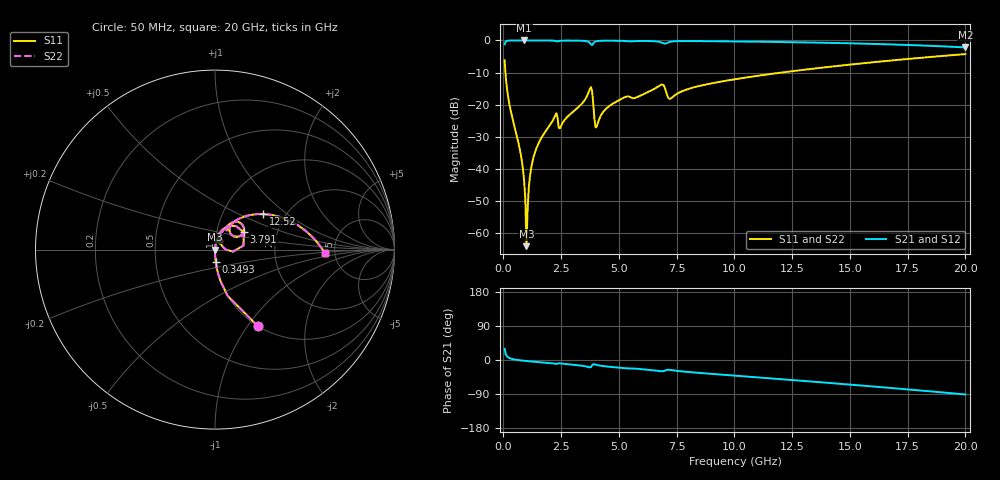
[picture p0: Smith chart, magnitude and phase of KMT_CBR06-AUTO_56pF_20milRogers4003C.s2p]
! Data measured by Modelithics Inc. support@modelithics.com 813-866-6335
! KEMET CBR06-AUTO 56pF, Pad Width= 0.851mm, Pad Length= 0.64mm, Pad Gap= 0.62mm, 20mil Rogers 4003C substrate Data, January 2022
# hz S ma R 50
! 2 Port Network Data from SP1.SP block
! freq  magS11  angS11  magS21  angS21  magS12  angS12  magS22  angS22
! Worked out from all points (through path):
!   401 points, 50 MHz to 20 GHz, reference 50 ohm
!   highest |S21| = 0.00 dB at 897.9 MHz (marker M1); lowest = -2.2 dB at 20 GHz (marker M2)
!   group delay of S21, straight-line fit = 12.8 ps
!   lowest |S11| = -64.0 dB at 997.6 MHz (marker M3), VSWR 1.00, Z = 50 - j0.0408 ohm
!   |S11| at or under -10 dB: 86.67 MHz to 12.03 GHz (11.95 GHz wide, 197 % of centre)
!   |S22| runs from -64.0 to -4.2 dB; largest |S21 - S12| = 0
!   S11 on the Smith chart (normalised r, x): 50 MHz: 1.00, -1.13; 349.2 MHz: 1.00, -0.14; 3.791 GHz: 1.35, +0.27; 12.52 GHz: 1.54, +0.69; 20 GHz: 4.15, -0.28
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5e7  0.4912 -60.7  0.8707 29.3  0.8707 29.3  0.4912 -60.7
3.4925e8  0.07109 -86.6  0.9972 3.1  0.9972 3.1  0.07109 -86.6
7.4825e8  0.01695 -89.6  0.9994 -1.1  0.9994 -1.1  0.01695 -89.6
8.97875e8  0.006417 -87.9  0.9995 -2.1  0.9995 -2.1  0.006417 -87.9
9.97625e8  0.0006298 -40.3  0.9995 -2.7  0.9995 -2.7  0.0006298 -40.3
1.097375e9  0.005117 80.8  0.9994 -3.3  0.9994 -3.3  0.005117 80.8
1.197125e9  0.01019 83.0  0.9993 -3.8  0.9993 -3.8  0.01019 83.0
1.296875e9  0.01499 83.4  0.9993 -4.4  0.9993 -4.4  0.01499 83.4
1.646e9  0.03066 82.4  0.9987 -6.2  0.9987 -6.2  0.03066 82.4
2.194625e9  0.06233 74.9  0.992 -9.5  0.992 -9.5  0.06233 74.9
2.493875e9  0.04681 71.5  0.9914 -9.4  0.9914 -9.4  0.04681 71.5
3.391625e9  0.1036 72.0  0.9893 -15.1  0.9893 -15.1  0.1036 72.0
3.790625e9  0.1873 31.0  0.868 -18.4  0.868 -18.4  0.1873 31.0
4.04e9  0.04577 44.9  0.9749 -13.1  0.9749 -13.1  0.04577 44.9
4.788125e9  0.1065 68.5  0.9896 -19.0  0.9896 -19.0  0.1065 68.5
6.73325e9  0.1957 52.6  0.9533 -29.3  0.9533 -29.3  0.1957 52.6
7.232e9  0.1243 46.0  0.9548 -26.3  0.9548 -26.3  0.1243 46.0
1.0025e10  0.2491 48.0  0.965 -41.3  0.965 -41.3  0.2491 48.0
1.251875e10  0.3329 36.5  0.9393 -52.9  0.9393 -52.9  0.3329 36.5
1.336662e10  0.3623 32.5  0.9282 -57.0  0.9282 -57.0  0.3623 32.5
1.670825e10  0.4846 15.9  0.8689 -73.5  0.8689 -73.5  0.4846 15.9
2e10  0.6131 -2.0  0.7784 -91.0  0.7784 -91.0  0.6131 -2.0
